PROGRAM MAIN
VAR
	eventTimeStamp									: Timestamp_Struct;	
	timeArray										: ARRAY [0..255] OF Timestamp_Struct;
	idx												: BYTE;
	
	ExtTimeLatch1									: T_DCTIME64:=0;
	ExtTimeLatch2									: T_DCTIME64:=0;
	UtcTimeValue1									: ULINT:=0;
	UtcTimeValue2									: ULINT:=0;
	
	
	OverrideUtcOffset_sec							: INT;	(*Use this field to set UTC Offset in seconds manually if Grandmaster does not provide valid UTC offset*)
	CurrentUtcOffset_nsec							: LINT;

	fbTimer											: TON;
	bRestartRdDiag									: BOOL;
	fbRdPtpDiag										: FB_GetPtpDiag;
	fbSyncCheck										: FB_EcExtSyncCheck64;
	fbFlanke										: R_Trig;
	CurrentUtcOffset1: INT;
	
	(*copy of *)
	DcToExtTimeOffset					 			: ULINT; 
	DcToTcTimeOffset 								: ULINT; 
END_VAR

DcToExtTimeOffset:=LINT_TO_ULINT(GVL.DcToExtTimeOffset);
DcToTcTimeOffset:=LINT_TO_ULINT(GVL.DcToTcTimeOffset);

(*Check Syncronisation*)
fbSyncCheck(
	nSyncWindow			:= 5000, (*5 us*)
	bNotConnected		:= GVL.bExternalDeviceNotConnected,
	DcToTcTimeOffset 	:= DcToTcTimeOffset,
	DcToExtTimeOffset 	:= DcToExtTimeOffset,
	ExtTime				:= GVL.ExtTime,
	IntTime				:= GVL.IntTime  );

IF NOT fbSyncCheck.bSynchronized THEN
	;(* ToDo: Handle SyncError ==> f. e. signal "Sync Error Event" to Application*)
ELSE
	(*CALCULATION OF EXTERNAL TIME - at beginning of task*)  
	ExtTimeLatch1													:=	F_GetCurExtTime64(DcToExtTimeOffset:=DcToExtTimeOffset, DcToTcTimeOffset:=DcToTcTimeOffset);
	(*As String: External time - at beginning of task*)
	eventTimeStamp.sCurExtTaskTime64								:=	DCTIME64_TO_STRING(ExtTimeLatch1);
	(*As String: External UTC time - at beginning of task*)
	eventTimeStamp.sCurExtTaskUtcTime64								:=	DCTIME64_TO_STRING(ULINT_TO_LINT(ExtTimeLatch1)-CurrentUtcOffset_nsec);
	(*As ULINT: External UTC time - at beginning of task*)
	UtcTimeValue1													:=	STRING_TO_DCTIME64(eventTimeStamp.sCurExtTaskUtcTime64);
	
	
	(*CALCULATION OF EXTERNAL TIME - actual Value*)
	ExtTimeLatch2													:=	F_ConvTcTimeToExtTime64(F_GetActualDcTime64(), DcToTcTimeOffset, DcToExtTimeOffset);
	(*As String: External time - actual value*)
	eventTimeStamp.sCurExtTime64									:=	DCTIME64_TO_STRING(ExtTimeLatch2);
	(*As String: External UTC time - actual value*)
	eventTimeStamp.sCurExtUtcTime64									:=	DCTIME64_TO_STRING(ULINT_TO_LINT(ExtTimeLatch2)-CurrentUtcOffset_nsec);
	(*As ULINT: External UTC time - actual value*)
	UtcTimeValue2													:=	STRING_TO_DCTIME64(eventTimeStamp.sCurExtUtcTime64);
	
	(*Trigger event generation on digital input terminal ==> EL1014 10us filter time*)
	fbFlanke(CLK:=GVL.bInput);
	IF fbFlanke.Q THEN
		timeArray[idx]:=eventTimeStamp;
		idx:=idx+1;
	END_IF
END_IF

(*Once per 1 Second -> Read Diag Object of EL6688 ==> CoE Index 0xFA80 to get current value of currentUtcOffset *)
fbRdPtpDiag(arrNetId:=GVL.EL6688NetId, nSlaveAddr:=GVL.EL6688SlaveAddr);
fbTimer(PT:=T#1S);
IF NOT fbTimer.Q THEN
	fbTimer(PT:=T#1S, IN:=TRUE);
ELSE
	bRestartRdDiag:=TRUE;
	fbTimer(PT:=T#1S, IN:=FALSE);
END_IF
IF bRestartRdDiag THEN
	fbRdPtpDiag(arrNetId:=GVL.EL6688NetId, nSlaveAddr:=GVL.EL6688SlaveAddr);
	IF NOT fbRdPtpDiag.bBusy THEN
		fbRdPtpDiag.bStart:=TRUE;
	ELSE
		fbRdPtpDiag.bStart:=FALSE;
		bRestartRdDiag:=FALSE;
		IF NOT fbRdPtpDiag.bErr THEN
			IF OverrideUtcOffset_sec <> 0 THEN
				CurrentUtcOffset_nsec:=INT_TO_LINT(OverrideUtcOffset_sec)*1000000000;
			ELSIF fbRdPtpDiag.Diag.CurrentUtcOffsetIsValid <> 0 THEN
				CurrentUtcOffset_nsec:=INT_TO_LINT(fbRdPtpDiag.Diag.CurrentUtcOffset)*1000000000;
			ELSE
				CurrentUtcOffset_nsec:=0;
			END_IF
		END_IF
	END_IF
END_IF

END_PROGRAM
